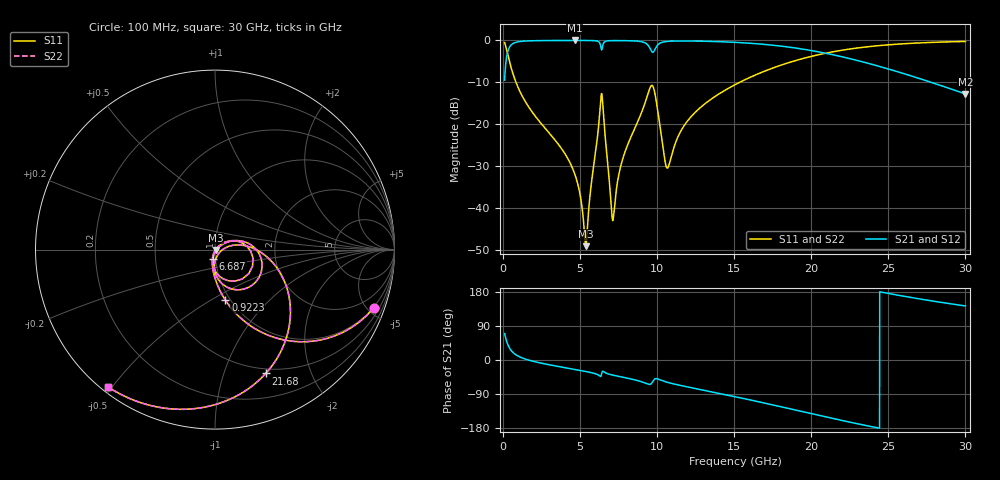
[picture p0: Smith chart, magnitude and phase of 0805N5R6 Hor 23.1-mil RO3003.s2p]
# GHz S MA R 50
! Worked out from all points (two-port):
!   3201 points, 100 MHz to 30 GHz, reference 50 ohm
!   highest |S21| = -0.03 dB at 4.65 GHz (marker M1); lowest = -12.8 dB at 30 GHz (marker M2)
!   |S21| within 3 dB of the highest: 280.5 MHz to 20.86 GHz (20.58 GHz wide, 195 % of centre)
!   lowest |S11| = -49.2 dB at 5.37 GHz (marker M3), VSWR 1.01, Z = 50.3 - j0.185 ohm
!   |S11| at or under -10 dB: 835.6 MHz to 15.37 GHz (14.53 GHz wide, 179 % of centre)
!   |S22| runs from -49.2 to -0.3 dB; largest |S21 - S12| = 0
!   S11 on the Smith chart (normalised r, x): 100 MHz: 0.95, -5.48; 922.2 MHz: 0.95, -0.58; 6.687 GHz: 0.97, -0.10; 21.68 GHz: 0.45, -1.39; 30 GHz: 0.02, -0.49
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0.1  0.9422 -20.1  0.3347 69.9  0.3347 69.9  0.9422 -20.1
0.47375  0.5095 -62.0  0.8599 27.9  0.8599 27.9  0.5095 -62.0
0.92225  0.2885 -78.3  0.9565 11.5  0.9565 11.5  0.2885 -78.3
4.650406  0.02532 -109.2  0.997 -24.9  0.997 -24.9  0.02532 -109.2
5.089563  0.0113 -103.0  0.9968 -28.1  0.9968 -28.1  0.0113 -103.0
5.369875  0.003475 -32.0  0.9963 -30.3  0.9963 -30.3  0.003475 -32.0
6.332281  0.19 1.4  0.8556 -43.2  0.8556 -43.2  0.19 1.4
6.472437  0.1683 -74.6  0.8738 -29.5  0.8738 -29.5  0.1683 -74.6
6.687344  0.05306 -103.2  0.9791 -34.7  0.9791 -34.7  0.05306 -103.2
7.005031  0.01131 -84.1  0.9918 -38.7  0.9918 -38.7  0.01131 -84.1
7.145187  0.00726 -20.4  0.9929 -40.1  0.9929 -40.1  0.00726 -20.4
7.771219  0.03876 35.0  0.9926 -45.5  0.9926 -45.5  0.03876 35.0
9.5185  0.2656 -12.8  0.813 -64.5  0.813 -64.5  0.2656 -12.8
9.770781  0.2684 -55.8  0.7315 -53.0  0.7315 -53.0  0.2684 -55.8
10.06978  0.1314 -89.1  0.8935 -50.6  0.8935 -50.6  0.1314 -89.1
10.68647  0.02996 -32.7  0.9727 -59.2  0.9727 -59.2  0.02996 -32.7
12.07869  0.1155 12.7  0.9823 -72.0  0.9823 -72.0  0.1155 12.7
15.05  0.2952 -8.4  0.9465 -96.8  0.9465 -96.8  0.2952 -8.4
20.03956  0.6458 -52.9  0.7531 -142.0  0.7531 -142.0  0.6458 -52.9
21.68406  0.7456 -67.7  0.6555 -156.9  0.6555 -156.9  0.7456 -67.7
25.01978  0.8851 -95.2  0.4537 175.5  0.4537 175.5  0.8851 -95.2
30  0.9701 -127.9  0.229 142.7  0.229 142.7  0.9701 -127.9
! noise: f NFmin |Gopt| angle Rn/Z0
0.1  0.0008299  0.9258  1.057  0.002481
3.417  0.006138  0.6971  19.67  0.003847
6.743  0.02384  0.8371  37.83  0.02773
10.06  0.07958  0.9261  55.25  0.1874
13.39  0.02507  0.7294  71.16  0.01235
16.7  0.02871  0.7179  85.73  0.01107
20.03  0.03581  0.7365  99.4  0.01173
23.35  0.04615  0.7681  112.4  0.01303
26.67  0.06156  0.8078  125  0.0148
30  0.08584  0.8517  137.6  0.01684
